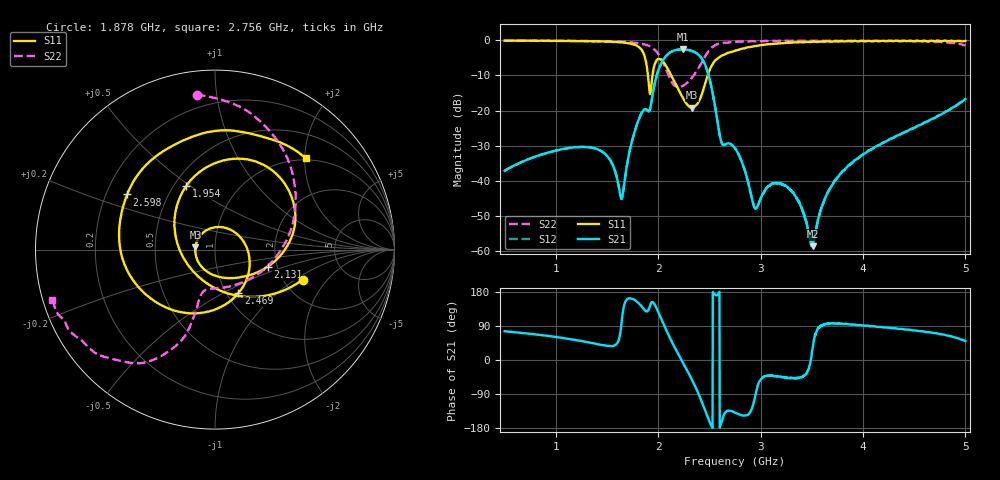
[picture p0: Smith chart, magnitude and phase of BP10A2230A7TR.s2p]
!Agilent Technologies,E8358A,US41080443,A.07.50.56
!Agilent E8358A: A.07.50.56
!Date: Tuesday, December 16, 2014 13:49:15
!Correction: S11(Full 2 Port(1,2))
!S21(Full 2 Port(1,2))
!S12(Full 2 Port(1,2))
!S22(Full 2 Port(1,2))
!S2P File: Measurements: S11, S21, S12, S22:
# Hz S  dB  R 50
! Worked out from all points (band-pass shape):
!   1601 points, 500 MHz to 5 GHz, reference 50 ohm
!   highest |S21| = -2.55 dB at 2.238 GHz (marker M1); lowest = -58.6 dB at 3.509 GHz (marker M2)
!   |S21| within 3 dB of the highest: 2.049 GHz to 2.434 GHz (385.2 MHz wide, 17.2 % of centre)
!   lowest |S11| = -19.2 dB at 2.328 GHz (marker M3), VSWR 1.25, Z = 40.2 + j1.01 ohm
!   |S11| at or under -10 dB: 1.9 GHz to 1.944 GHz (44.17 MHz wide, 2.3 % of centre); 2.127 GHz to 2.482 GHz (354.3 MHz wide, 15.4 % of centre)
!   |S22| runs from -13.4 to 0.0 dB; largest |S21 - S12| = 0.0038
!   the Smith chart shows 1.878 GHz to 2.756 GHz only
!   S11 on the Smith chart (normalised r, x): 1.878 GHz: 2.53, -1.15; 1.954 GHz: 0.58, +0.48; 2.131 GHz: 1.78, -0.38; 2.469 GHz: 1.13, -0.60; 2.598 GHz: 0.29, +0.27; 2.756 GHz: 0.96, +2.02
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5e8  -0.08 162.4  -37.13 76.0  -37.14 76.1  -0.06 172.9
1.250938e9  -0.20 125.6  -30.31 50.1  -30.35 50.3  -0.15 154.9
1.641875e9  -0.60 82.8  -45.08 97.0  -45.18 96.9  -0.42 132.3
1.776875e9  -1.33 48.7  -25.28 157.2  -25.34 157.2  -0.72 116.5
1.878125e9  -5.75 -19.0  -19.61 129.2  -19.59 129.2  -1.22 96.7
1.954062e9  -8.21 114.5  -14.00 150.9  -14.04 150.8  -2.33 71.8
2.001875e9  -5.29 60.3  -8.49 125.6  -8.51 125.7  -3.88 50.0
2.13125e9  -10.22 -18.1  -3.17 48.9  -3.19 49.0  -11.80 -38.4
2.238125e9  -16.24 -80.9  -2.55 -5.6  -2.56 -5.6  -12.96 -99.8
2.328125e9  -19.19 173.5  -3.00 -51.2  -3.03 -51.2  -10.70 -107.7
2.46875e9  -11.18 -62.1  -7.76 -141.0  -7.79 -140.9  -4.05 -114.8
2.598125e9  -4.76 147.9  -26.59 179.8  -26.61 179.6  -0.97 -143.9
2.75e9  -2.92 48.2  -30.68 -139.1  -30.75 -138.5  -0.48 -162.5
2.755625e9  -2.89 45.2  -30.96 -139.7  -30.97 -139.4  -0.46 -162.9
2.944062e9  -1.62 -26.3  -47.78 -98.8  -47.82 -98.3  -0.29 -176.5
3.07625e9  -1.12 -58.0  -41.50 -42.0  -41.57 -41.2  -0.23 177.3
3.318125e9  -0.58 -94.7  -43.40 -47.3  -43.35 -47.7  -0.06 169.2
3.500938e9  -0.42 -112.1  -57.66 20.2  -57.46 15.8  -0.15 164.6
3.509375e9  -0.39 -112.9  -58.61 33.8  -57.56 32.8  -0.10 164.5
3.72875e9  -0.29 -128.9  -39.69 95.7  -39.84 96.7  -0.04 159.7
4.251875e9  -0.09 -151.9  -28.26 85.3  -28.36 85.4  -0.19 150.5
5e9  -0.15 -172.3  -16.69 50.0  -16.73 50.1  -1.43 107.3
